(* Logix 5000 AddOnInstructionDefinition export Banner_IC70_Param_v4; software revision 33.03 *)

TYPE Banner_IC70_16P_Config_v4 :
STRUCT
   IO_Selection : INT;   // 0=NPN, 1=PNP
   Delay_Mode : INT;   // 0=Disabled,1=On Off Delay, 2=On OneShot, 3=Off OneShot, 4=On Pulse Stretcher, 5=Off Pulse Stretcher, 6=Totalizer, 7=Retriggerable On OneShot, 8=Retriggerable Off OneShot.
   Delay_Timer1 : DINT;
   Delay_Timer2 : DINT;
   Mirroring_Enable : SINT;   // 0=Disabled, 1=Enabled
   Mirroring_Channel : SINT;   // 0=C1, 1=C2, 2=C3, 3=C4, 4=C5, 5=C6, 6=C7, 7=C8, 8=C9, 9=C10, 10=C11, 11=C12, 12=C13, 13=C14, 14=C15, 15=C16
   Mirroring_Inversion : SINT;   // 0=Not Inverted, 1=Inverted
END_STRUCT
END_TYPE

TYPE Banner_IC70_16P_Direcrt_Param_v4 :
STRUCT
   Master_Cycle_Time : INT;
   Min_Cycle_Time : INT;
   M_Sequence_Capability : INT;
   IO_Link_Version_ID : INT;
   Process_Data_Input_Length : INT;
   Process_Data_Output_Length : INT;
   Combined_Vendor_ID : DINT;   // IO-Link Vendor ID
   Vendor_ID1 : INT;
   Vendor_ID2 : INT;
   Combined_Device_ID : DINT;   // IO-Link Device ID
   Device_ID1 : INT;
   Device_ID2 : INT;
   Device_ID3 : INT;
END_STRUCT
END_TYPE

TYPE Banner_IC70_16P_IO_Metrics_v4 :
STRUCT
   Count : DINT;
   Duration : DINT;
   Events_Per_Minute : DINT;
   Totalizer : DINT;
END_STRUCT
END_TYPE

TYPE Banner_IC70_16P_RD_v4 :   // UDT that stores the Write Data for a IC70-16P-K.
STRUCT
   Direct_Parameters : Banner_IC70_16P_Direcrt_Param_v4;
   Serial_Number : STRING;
   All_Time_Run_Time : DINT;   // Run Counter in 1/4 hr increments
   IO_Metrics : Banner_IC70_16P_IO_Metrics_v4[17];
END_STRUCT
END_TYPE

TYPE Banner_IC70_16P_SMR_Port_v4 :
STRUCT
   Reset : SINT;   // 0 = Normal setting, 1 = Reset metrics.
   Reset_Count : DINT;   // Value that Counter is set to when a Reset Metrics operation is activated.
END_STRUCT
END_TYPE

TYPE Banner_IC70_16P_v4 :   // All of the parameters for a IC70-16P.
STRUCT
   Initial_Global_Read : BOOL;   // Determines if all of the IO-Link data has been read into the PLC yet
   Command : INT;   // Value placed in here will activate a read or write to a specifc IO-Link Index
   Read : Banner_IC70_16P_RD_v4;   // Read Only Data
   Write : Banner_IC70_16P_WD_v4;   // Write Data
   Reset : BOOL;   // Resets AOI. This will force a complete parameter read of the sensor.
END_STRUCT
END_TYPE

TYPE Banner_IC70_16P_WD_v4 :   // UDT that stores the Write Data for a IC70-16P-K.
STRUCT
   System_Command : INT;   // See IODD file for list of commands that can be activated via the System Command interface
   Parameter_Access_Lock : SINT;   // Write access to all parameters is prohibited while value is 1. Only this parameter can be adjusted when value is 1.
   Data_Storage_Lock : SINT;   // Automatic data storage is disabled when this value is equal to 1. Read access is not affected.
   Local_Parameterization_Lock : SINT;   // Parameterization via local control elements on device is disabled.
   Local_User_Interface_Lock : SINT;   // Operation of local user interface is disabled.
   Resettable_Run_Time : DINT;   // Run Counter in 1/4 hr increments
   All_Time_Run_Time_Event_Time : DINT;   // Event Time in 1/4 hr increments
   Resettable_Run_Time_Event_Time : DINT;   // Event Time in 1/4 hour increments
   SMR : Banner_IC70_16P_SMR_Port_v4[17];   // Selectable Metric Reset.
   Channel_Config : Banner_IC70_16P_Config_v4[17];
END_STRUCT
END_TYPE

TYPE Banner_IOL_Port_v4 :   // UDT that has all of the data items necessary to communicate with a specific Port on a IO-Link Master
STRUCT
   Port_Controlled : INT;   // Each bit represents a port on an IO-Link Master. Set to 1 to tell AOI to control that port.
   Port_Activate : INT;   // Each bit represents a port on an IO-Link Master. When ON that port will process any commands in queue.
   Port_Read : INT;   // Each bit represents a port on an IO-Link Master. Used to determine when device AOI has requested a Read command.
   Port_Write : INT;   // Each bit represents a port on an IO-Link Master. Used to determine when device AOI has requested a Write command.
   Port_RW_Complete : INT;   // Each bit represents a port on an IO-Link Master. Tells device AOI that Read or Write request has been completed.
   Port_Device_Read : INT;
   Data_Transfer : SINT[190];   // Array to transfer data from IO-Master to device AOIs.
END_STRUCT
END_TYPE

ADD_ON_INSTRUCTION Banner_IC70_Param_v4   (* revision 4.4, vendor Banner Engineering *)
// AOI to read and write parameter data to an IC70-16P-K IO-Link Hub.
// Revision note:
// Added R130C.
VAR_IN_OUT
   Hub : Banner_IC70_16P_v4; {required}
   Port_Data : Banner_IOL_Port_v4; {required}
END_VAR
VAR_INPUT
   Port : INT; {required}
END_VAR
VAR
   Control : DINT; {access None}
   Global_Read_Command_Value : INT; {access None}
   Global_Write_Command_Value : INT; {access None}
   Command_Being_Processed : BOOL; {access None}
   Update_Archive : BOOL; {access None}
   Index_Write_Inprocess : INT; {access None}
   Index_Write_Control : INT; {access None}
   Temp_Excess_Gain : DINT; {access None}
   Inprocess_Index : DINT; {access None}
   Index2 : SINT; {access None}
   Index1 : SINT; {access None}
   Index4 : SINT; {access None}
   Index3 : SINT; {access None}
   Index6 : SINT; {access None}
   Index5 : SINT; {access None}
   Index7 : SINT; {access None}
END_VAR

ROUTINE Logic   (* ladder *)
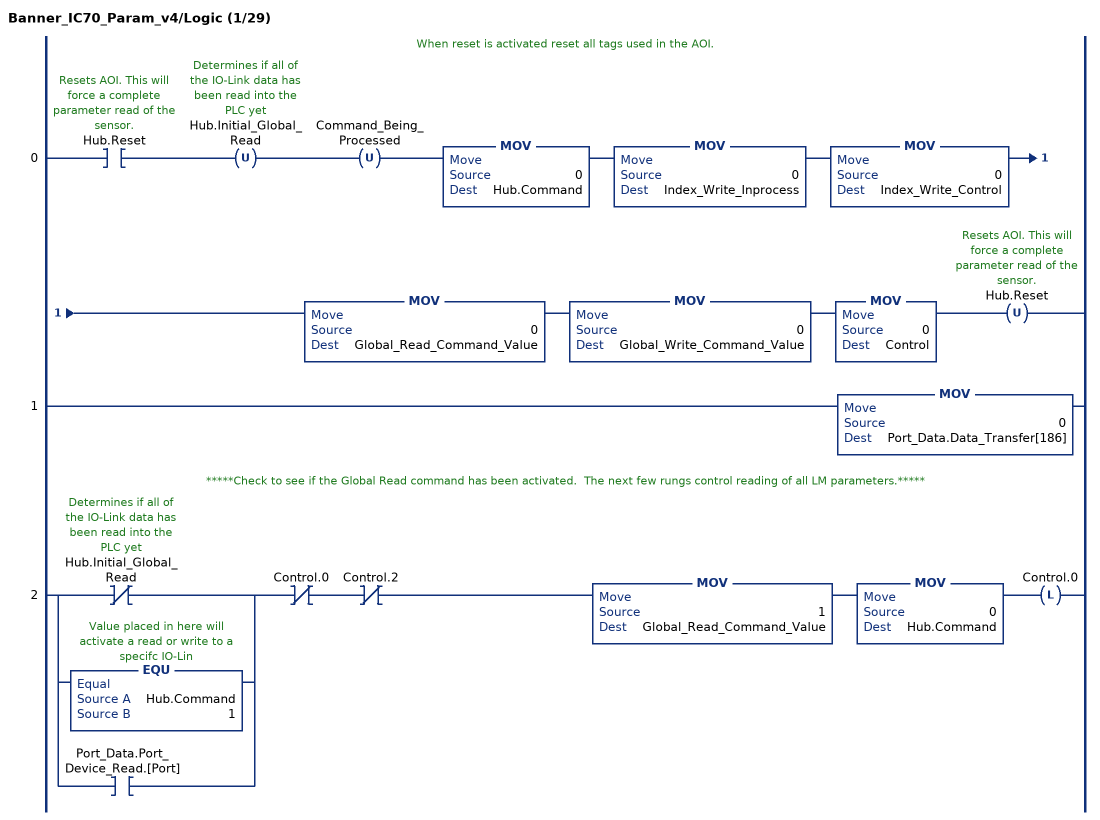
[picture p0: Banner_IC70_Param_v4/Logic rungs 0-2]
   // When reset is activated reset all tags used in the AOI.
   0: XIC(Hub.Reset)OTU(Hub.Initial_Global_Read)OTU(Command_Being_Processed)MOV(0,Hub.Command)MOV(0,Index_Write_Inprocess)MOV(0,Index_Write_Control)MOV(0,Global_Read_Command_Value)MOV(0,Global_Write_Command_Value)MOV(0,Control)OTU(Hub.Reset);
   1: MOV(0,Port_Data.Data_Transfer[186]);
   // *****Check to see if the Global Read command has been activated.  The next few rungs control reading of all LM parameters.*****
   2: [XIO(Hub.Initial_Global_Read) ,EQU(Hub.Command,1) ,XIC(Port_Data.Port_Device_Read.[Port]) ]XIO(Control.0)XIO(Control.2)MOV(1,Global_Read_Command_Value)MOV(0,Hub.Command)OTL(Control.0);
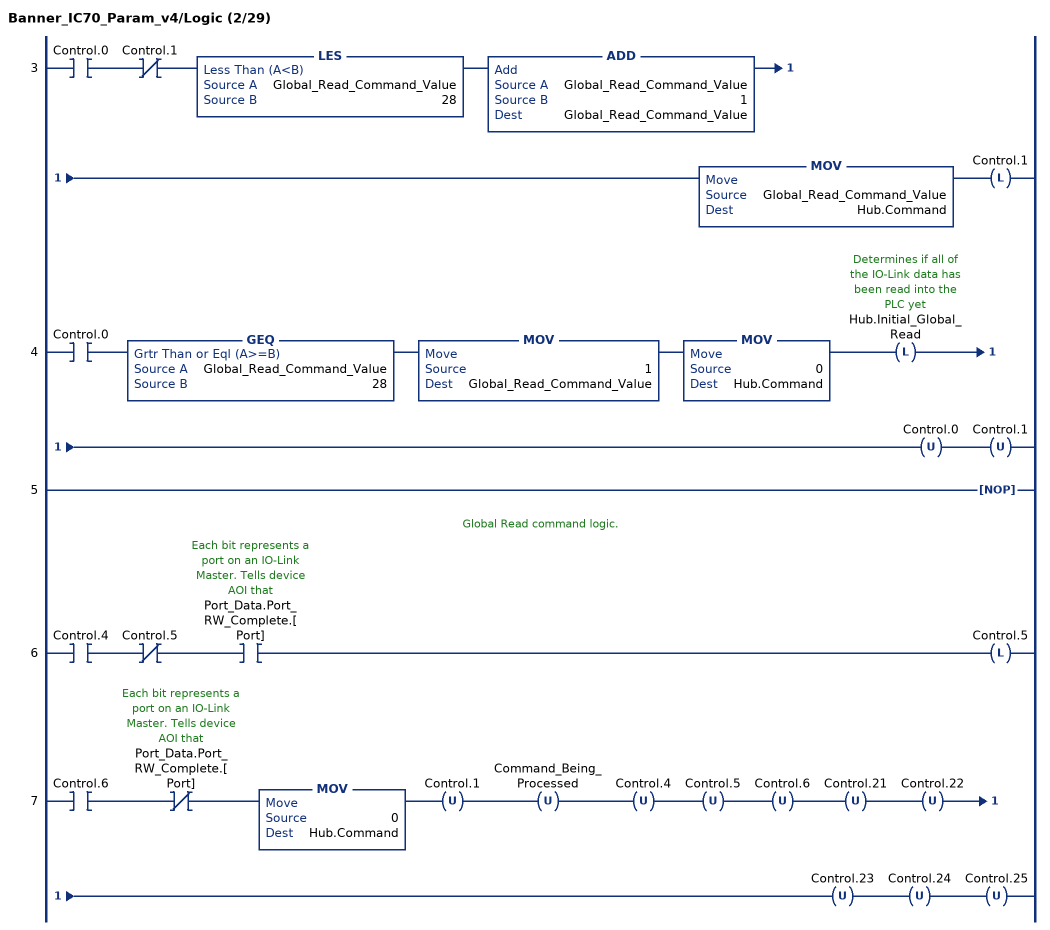
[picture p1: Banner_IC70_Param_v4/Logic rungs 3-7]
   3: XIC(Control.0)XIO(Control.1)LES(Global_Read_Command_Value,28)ADD(Global_Read_Command_Value,1,Global_Read_Command_Value)MOV(Global_Read_Command_Value,Hub.Command)OTL(Control.1);
   4: XIC(Control.0)GEQ(Global_Read_Command_Value,28)MOV(1,Global_Read_Command_Value)MOV(0,Hub.Command)OTL(Hub.Initial_Global_Read)OTU(Control.0)OTU(Control.1);
   5: NOP();
   // Global Read command logic.
   6: XIC(Control.4)XIO(Control.5)XIC(Port_Data.Port_RW_Complete.[Port])OTL(Control.5);
   7: XIC(Control.6)XIO(Port_Data.Port_RW_Complete.[Port])MOV(0,Hub.Command)OTU(Control.1)OTU(Command_Being_Processed)OTU(Control.4)OTU(Control.5)OTU(Control.6)OTU(Control.21)OTU(Control.22)OTU(Control.23)OTU(Control.24)OTU(Control.25);
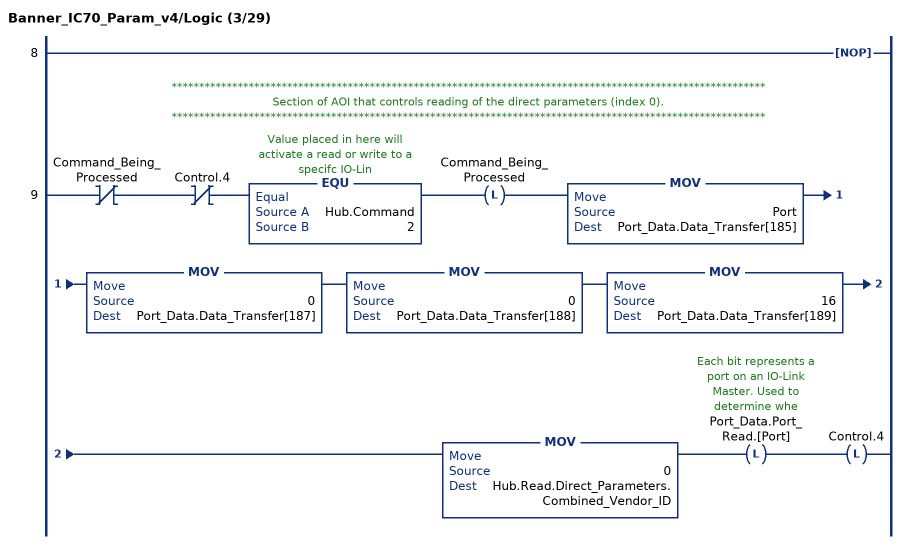
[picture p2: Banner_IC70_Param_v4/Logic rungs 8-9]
   8: NOP();
   // ************************************************************************************************************
   // Section of AOI that controls reading of the direct parameters (index 0).
   // ************************************************************************************************************
   9: XIO(Command_Being_Processed)XIO(Control.4)EQU(Hub.Command,2)OTL(Command_Being_Processed)MOV(Port,Port_Data.Data_Transfer[185])MOV(0,Port_Data.Data_Transfer[187])MOV(0,Port_Data.Data_Transfer[188])MOV(16,Port_Data.Data_Transfer[189])MOV(0,Hub.Read.Direct_Parameters.Combined_Vendor_ID)OTL(Port_Data.Port_Read.[Port])OTL(Control.4);
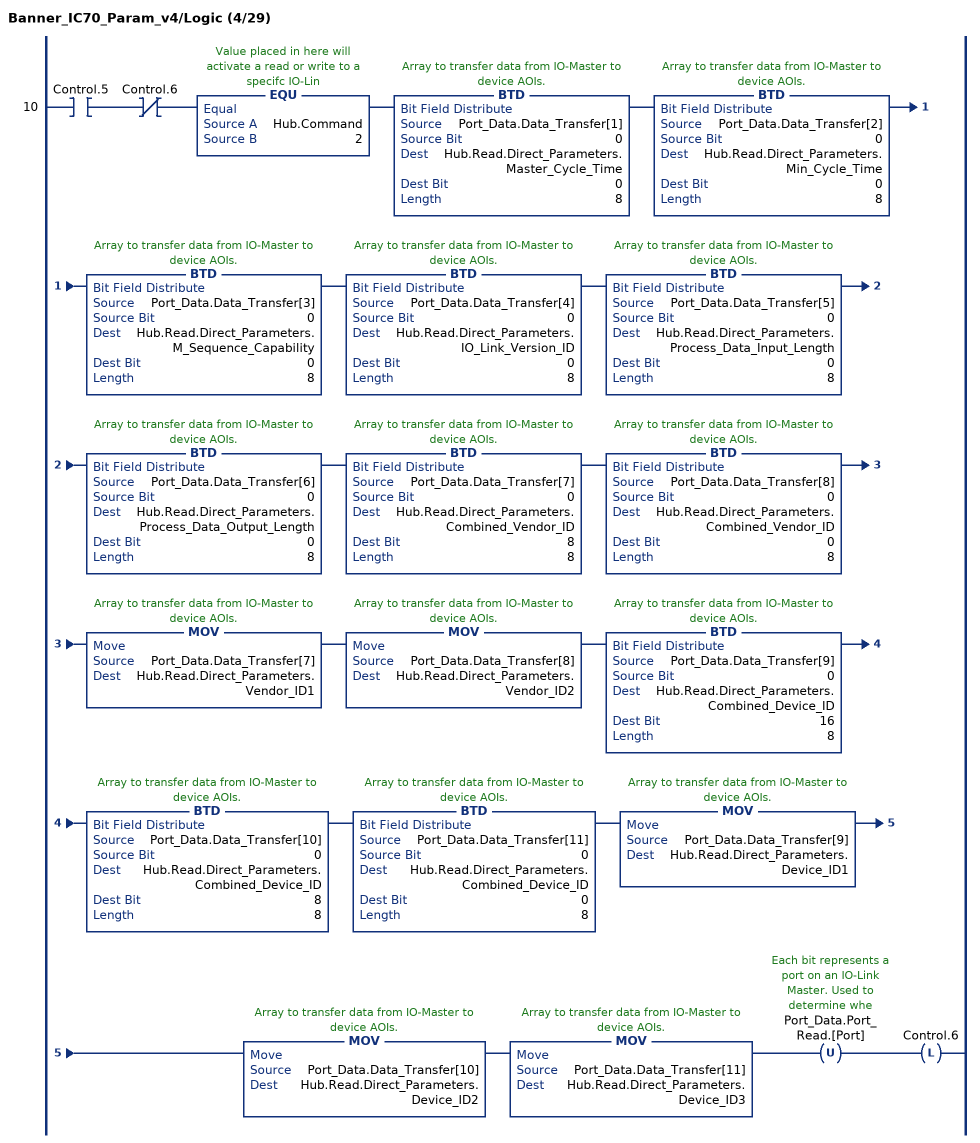
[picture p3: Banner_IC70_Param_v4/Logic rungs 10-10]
   10: XIC(Control.5)XIO(Control.6)EQU(Hub.Command,2)BTD(Port_Data.Data_Transfer[1],0,Hub.Read.Direct_Parameters.Master_Cycle_Time,0,8)BTD(Port_Data.Data_Transfer[2],0,Hub.Read.Direct_Parameters.Min_Cycle_Time,0,8)BTD(Port_Data.Data_Transfer[3],0,Hub.Read.Direct_Parameters.M_Sequence_Capability,0,8)BTD(Port_Data.Data_Transfer[4],0,Hub.Read.Direct_Parameters.IO_Link_Version_ID,0,8)BTD(Port_Data.Data_Transfer[5],0,Hub.Read.Direct_Parameters.Process_Data_Input_Length,0,8)BTD(Port_Data.Data_Transfer[6],0,Hub.Read.Direct_Parameters.Process_Data_Output_Length,0,8)BTD(Port_Data.Data_Transfer[7],0,Hub.Read.Direct_Parameters.Combined_Vendor_ID,8,8)BTD(Port_Data.Data_Transfer[8],0,Hub.Read.Direct_Parameters.Combined_Vendor_ID,0,8)MOV(Port_Data.Data_Transfer[7],Hub.Read.Direct_Parameters.Vendor_ID1)MOV(Port_Data.Data_Transfer[8],Hub.Read.Direct_Parameters.Vendor_ID2)BTD(Port_Data.Data_Transfer[9],0,Hub.Read.Direct_Parameters.Combined_Device_ID,16,8)BTD(Port_Data.Data_Transfer[10],0,Hub.Read.Direct_Parameters.Combined_Device_ID,8,8)BTD(Port_Data.Data_Transfer[11],0,Hub.Read.Direct_Parameters.Combined_Device_ID,0,8)MOV(Port_Data.Data_Transfer[9],Hub.Read.Direct_Parameters.Device_ID1)MOV(Port_Data.Data_Transfer[10],Hub.Read.Direct_Parameters.Device_ID2)MOV(Port_Data.Data_Transfer[11],Hub.Read.Direct_Parameters.Device_ID3)OTU(Port_Data.Port_Read.[Port])OTL(Control.6);
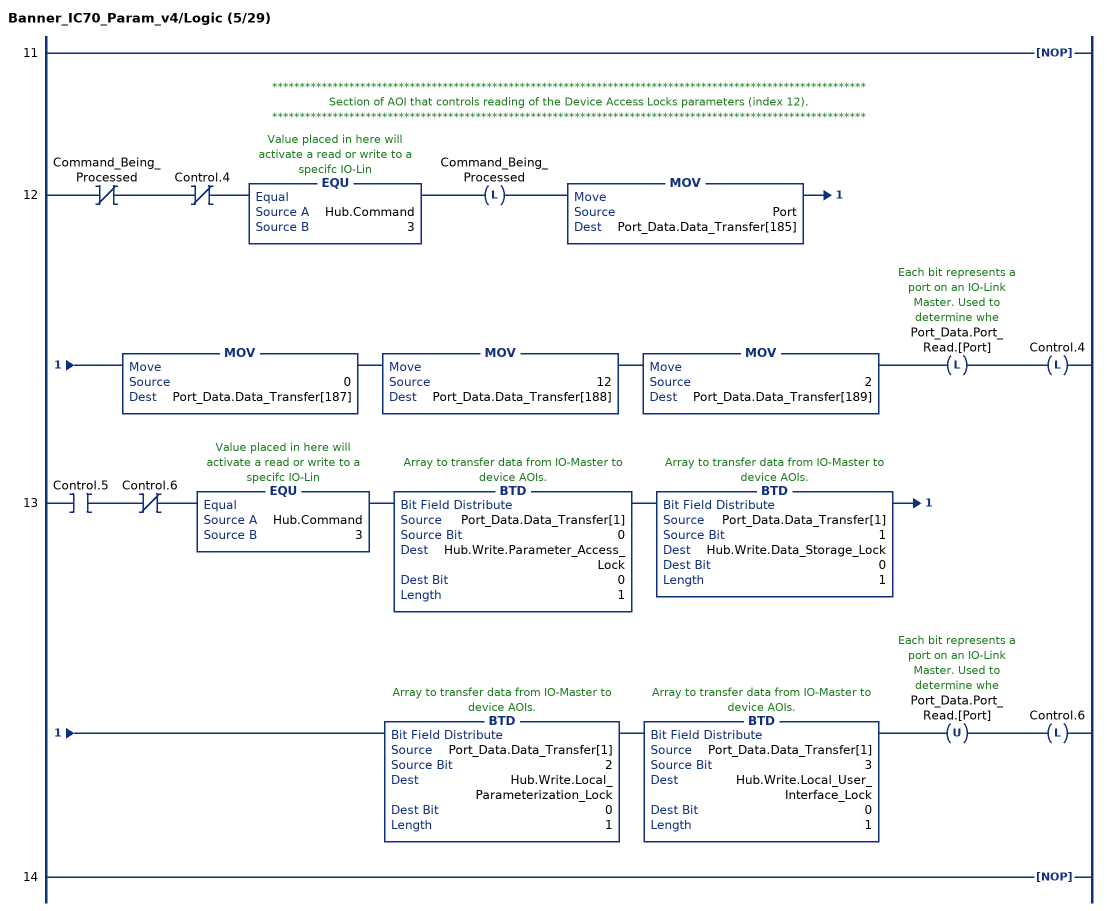
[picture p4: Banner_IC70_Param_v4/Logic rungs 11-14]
   11: NOP();
   // ************************************************************************************************************
   // Section of AOI that controls reading of the Device Access Locks parameters (index 12).
   // ************************************************************************************************************
   12: XIO(Command_Being_Processed)XIO(Control.4)EQU(Hub.Command,3)OTL(Command_Being_Processed)MOV(Port,Port_Data.Data_Transfer[185])MOV(0,Port_Data.Data_Transfer[187])MOV(12,Port_Data.Data_Transfer[188])MOV(2,Port_Data.Data_Transfer[189])OTL(Port_Data.Port_Read.[Port])OTL(Control.4);
   13: XIC(Control.5)XIO(Control.6)EQU(Hub.Command,3)BTD(Port_Data.Data_Transfer[1],0,Hub.Write.Parameter_Access_Lock,0,1)BTD(Port_Data.Data_Transfer[1],1,Hub.Write.Data_Storage_Lock,0,1)BTD(Port_Data.Data_Transfer[1],2,Hub.Write.Local_Parameterization_Lock,0,1)BTD(Port_Data.Data_Transfer[1],3,Hub.Write.Local_User_Interface_Lock,0,1)OTU(Port_Data.Port_Read.[Port])OTL(Control.6);
   14: NOP();
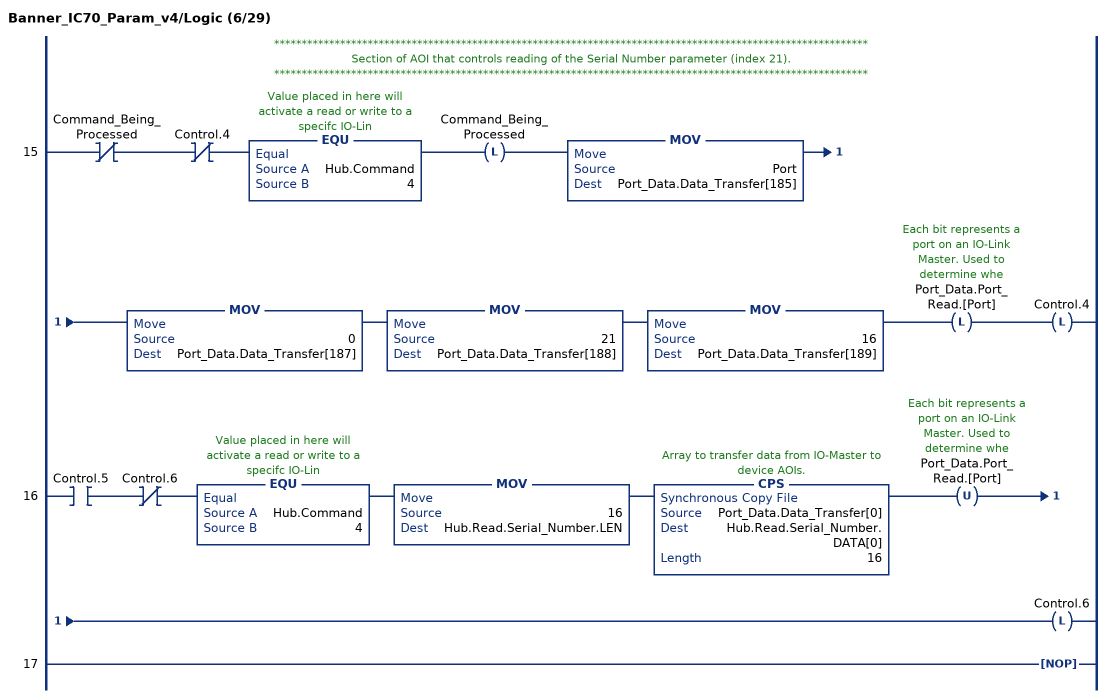
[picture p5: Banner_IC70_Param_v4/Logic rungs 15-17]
   // ************************************************************************************************************
   // Section of AOI that controls reading of the Serial Number parameter (index 21).
   // ************************************************************************************************************
   15: XIO(Command_Being_Processed)XIO(Control.4)EQU(Hub.Command,4)OTL(Command_Being_Processed)MOV(Port,Port_Data.Data_Transfer[185])MOV(0,Port_Data.Data_Transfer[187])MOV(21,Port_Data.Data_Transfer[188])MOV(16,Port_Data.Data_Transfer[189])OTL(Port_Data.Port_Read.[Port])OTL(Control.4);
   16: XIC(Control.5)XIO(Control.6)EQU(Hub.Command,4)MOV(16,Hub.Read.Serial_Number.LEN)CPS(Port_Data.Data_Transfer[0],Hub.Read.Serial_Number.DATA[0],16)OTU(Port_Data.Port_Read.[Port])OTL(Control.6);
   17: NOP();
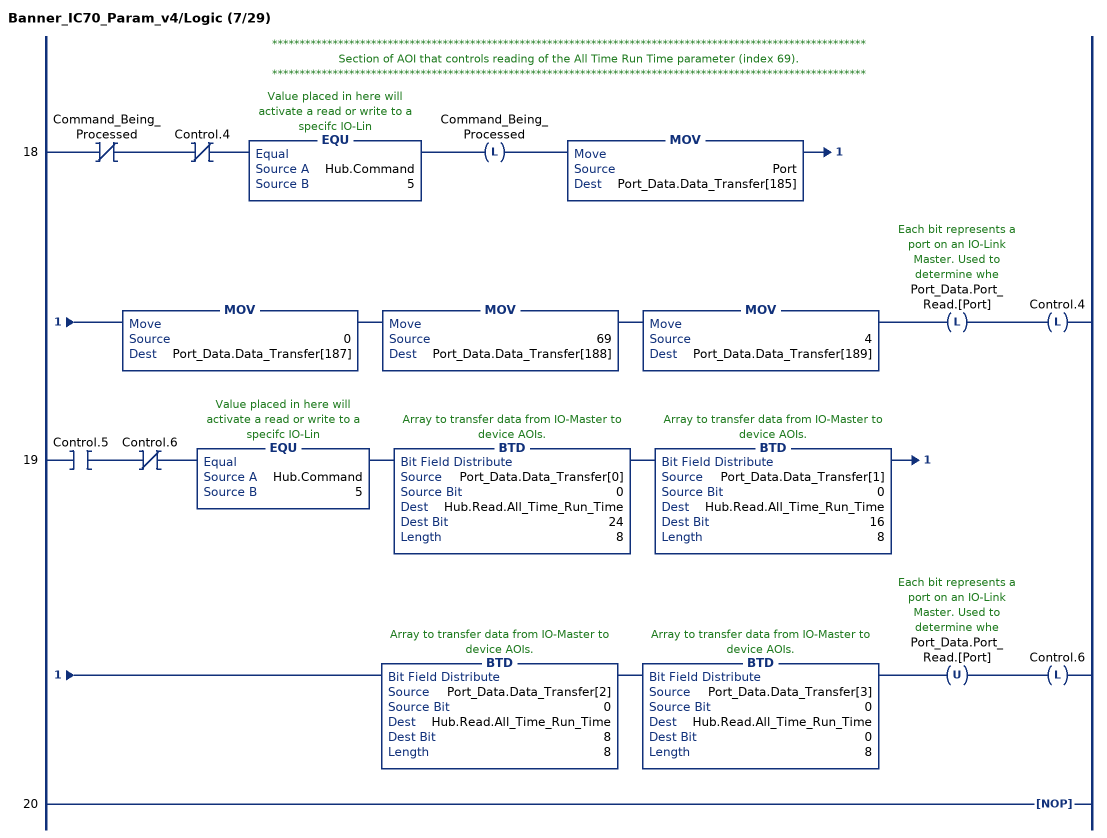
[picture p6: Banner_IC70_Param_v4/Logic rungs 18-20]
   // ************************************************************************************************************
   // Section of AOI that controls reading of the All Time Run Time parameter (index 69).
   // ************************************************************************************************************
   18: XIO(Command_Being_Processed)XIO(Control.4)EQU(Hub.Command,5)OTL(Command_Being_Processed)MOV(Port,Port_Data.Data_Transfer[185])MOV(0,Port_Data.Data_Transfer[187])MOV(69,Port_Data.Data_Transfer[188])MOV(4,Port_Data.Data_Transfer[189])OTL(Port_Data.Port_Read.[Port])OTL(Control.4);
   19: XIC(Control.5)XIO(Control.6)EQU(Hub.Command,5)BTD(Port_Data.Data_Transfer[0],0,Hub.Read.All_Time_Run_Time,24,8)BTD(Port_Data.Data_Transfer[1],0,Hub.Read.All_Time_Run_Time,16,8)BTD(Port_Data.Data_Transfer[2],0,Hub.Read.All_Time_Run_Time,8,8)BTD(Port_Data.Data_Transfer[3],0,Hub.Read.All_Time_Run_Time,0,8)OTU(Port_Data.Port_Read.[Port])OTL(Control.6);
   20: NOP();
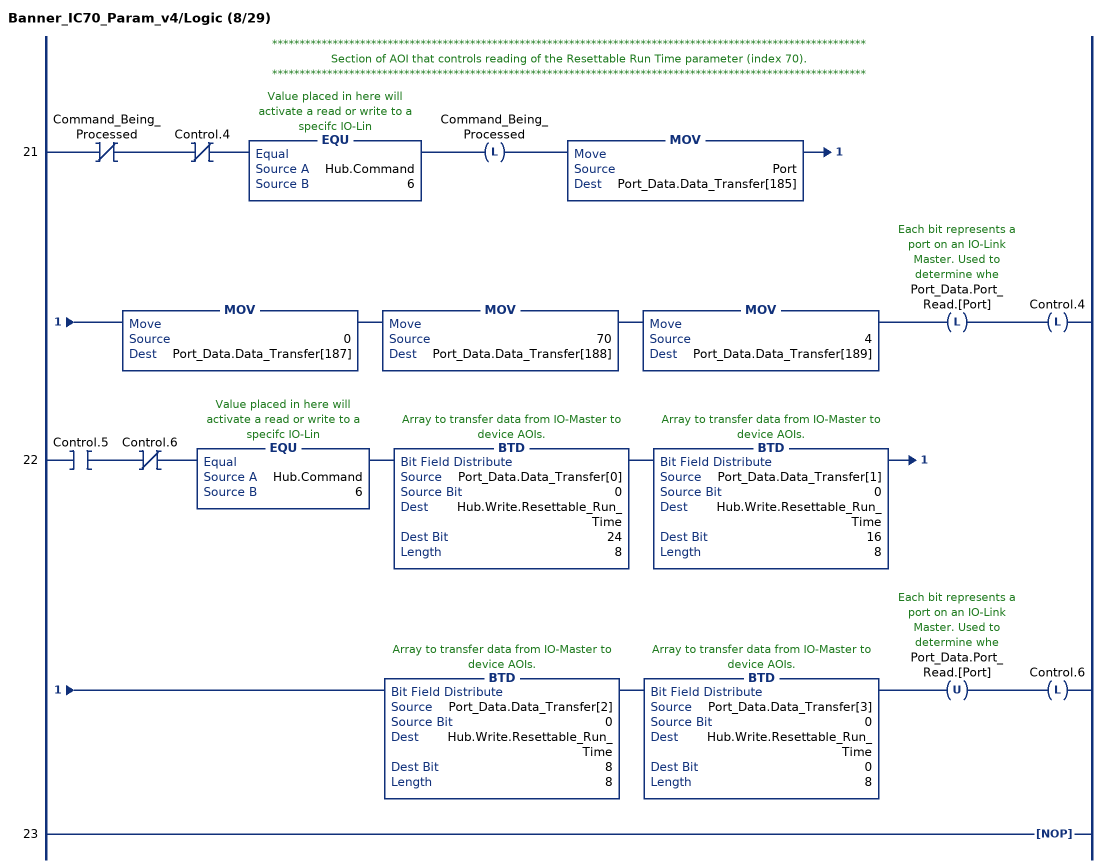
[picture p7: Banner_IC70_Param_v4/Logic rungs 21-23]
   // ************************************************************************************************************
   // Section of AOI that controls reading of the Resettable Run Time parameter (index 70).
   // ************************************************************************************************************
   21: XIO(Command_Being_Processed)XIO(Control.4)EQU(Hub.Command,6)OTL(Command_Being_Processed)MOV(Port,Port_Data.Data_Transfer[185])MOV(0,Port_Data.Data_Transfer[187])MOV(70,Port_Data.Data_Transfer[188])MOV(4,Port_Data.Data_Transfer[189])OTL(Port_Data.Port_Read.[Port])OTL(Control.4);
   22: XIC(Control.5)XIO(Control.6)EQU(Hub.Command,6)BTD(Port_Data.Data_Transfer[0],0,Hub.Write.Resettable_Run_Time,24,8)BTD(Port_Data.Data_Transfer[1],0,Hub.Write.Resettable_Run_Time,16,8)BTD(Port_Data.Data_Transfer[2],0,Hub.Write.Resettable_Run_Time,8,8)BTD(Port_Data.Data_Transfer[3],0,Hub.Write.Resettable_Run_Time,0,8)OTU(Port_Data.Port_Read.[Port])OTL(Control.6);
   23: NOP();
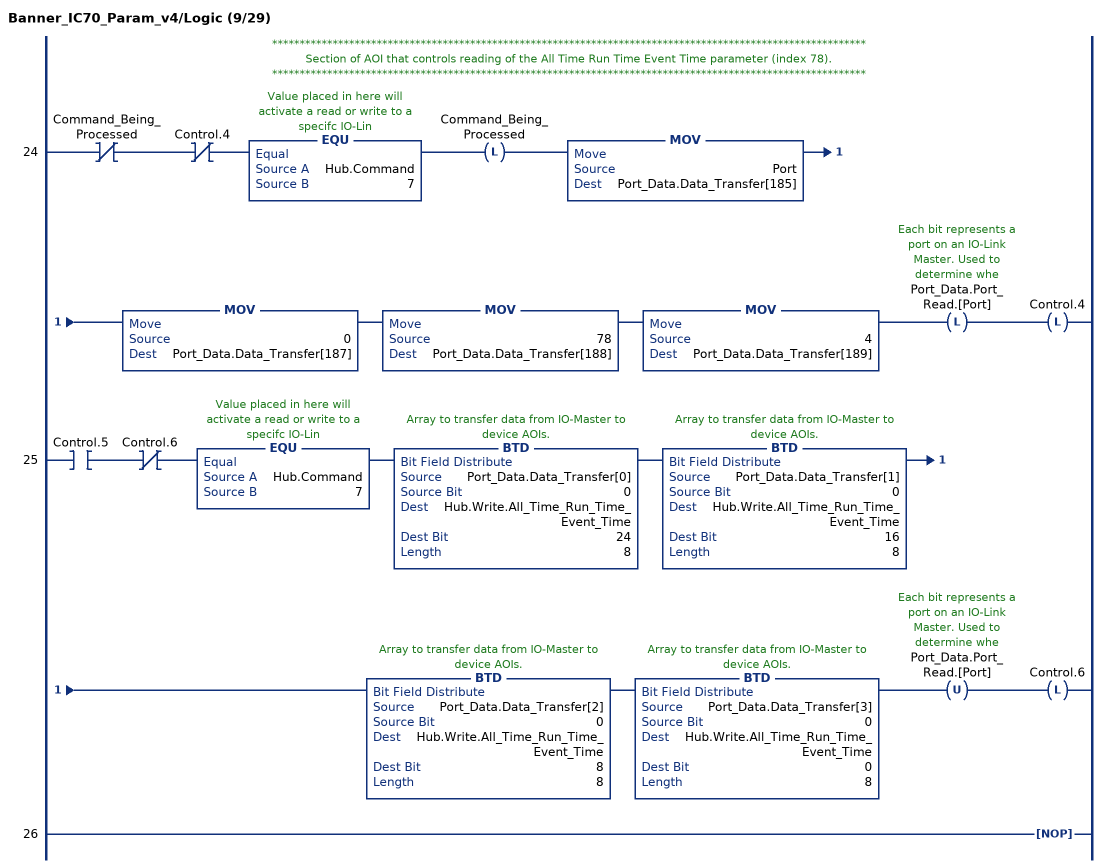
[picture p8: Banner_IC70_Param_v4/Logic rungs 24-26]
   // ************************************************************************************************************
   // Section of AOI that controls reading of the All Time Run Time Event Time parameter (index 78).
   // ************************************************************************************************************
   24: XIO(Command_Being_Processed)XIO(Control.4)EQU(Hub.Command,7)OTL(Command_Being_Processed)MOV(Port,Port_Data.Data_Transfer[185])MOV(0,Port_Data.Data_Transfer[187])MOV(78,Port_Data.Data_Transfer[188])MOV(4,Port_Data.Data_Transfer[189])OTL(Port_Data.Port_Read.[Port])OTL(Control.4);
   25: XIC(Control.5)XIO(Control.6)EQU(Hub.Command,7)BTD(Port_Data.Data_Transfer[0],0,Hub.Write.All_Time_Run_Time_Event_Time,24,8)BTD(Port_Data.Data_Transfer[1],0,Hub.Write.All_Time_Run_Time_Event_Time,16,8)BTD(Port_Data.Data_Transfer[2],0,Hub.Write.All_Time_Run_Time_Event_Time,8,8)BTD(Port_Data.Data_Transfer[3],0,Hub.Write.All_Time_Run_Time_Event_Time,0,8)OTU(Port_Data.Port_Read.[Port])OTL(Control.6);
   26: NOP();
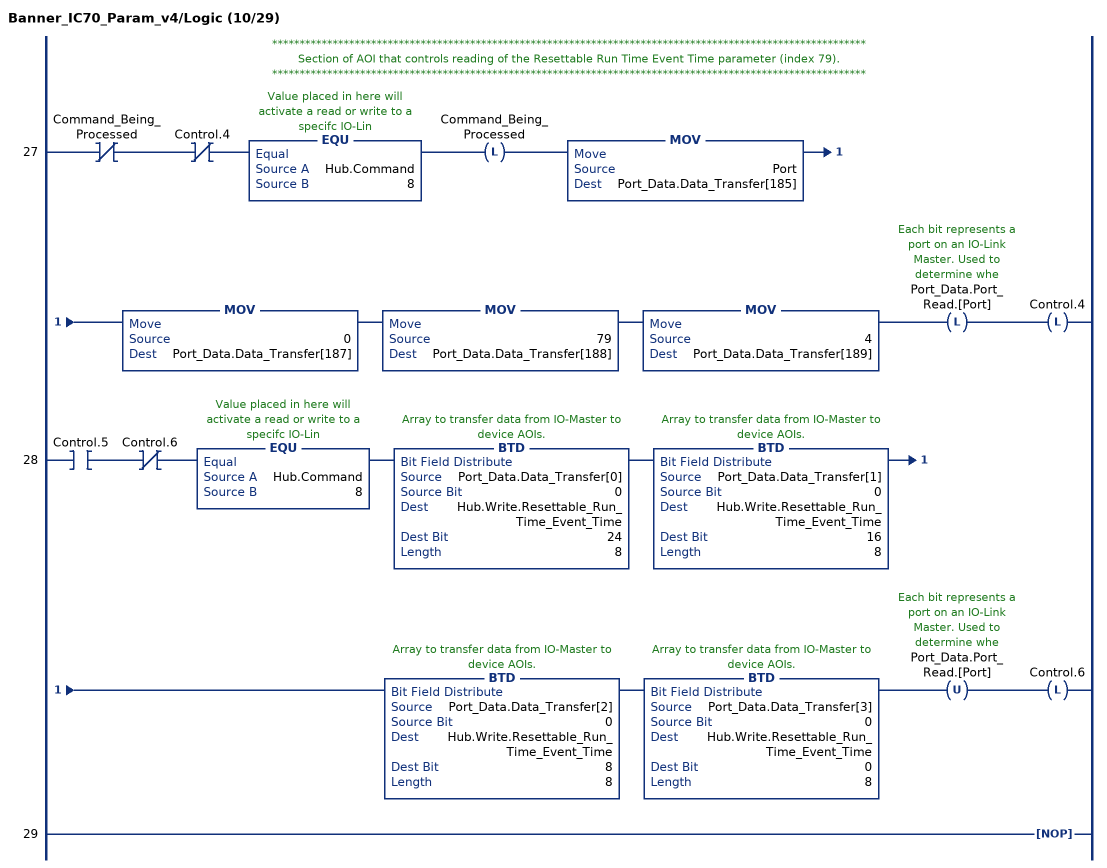
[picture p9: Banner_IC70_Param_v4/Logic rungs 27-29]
   // ************************************************************************************************************
   // Section of AOI that controls reading of the Resettable Run Time Event Time parameter (index 79).
   // ************************************************************************************************************
   27: XIO(Command_Being_Processed)XIO(Control.4)EQU(Hub.Command,8)OTL(Command_Being_Processed)MOV(Port,Port_Data.Data_Transfer[185])MOV(0,Port_Data.Data_Transfer[187])MOV(79,Port_Data.Data_Transfer[188])MOV(4,Port_Data.Data_Transfer[189])OTL(Port_Data.Port_Read.[Port])OTL(Control.4);
   28: XIC(Control.5)XIO(Control.6)EQU(Hub.Command,8)BTD(Port_Data.Data_Transfer[0],0,Hub.Write.Resettable_Run_Time_Event_Time,24,8)BTD(Port_Data.Data_Transfer[1],0,Hub.Write.Resettable_Run_Time_Event_Time,16,8)BTD(Port_Data.Data_Transfer[2],0,Hub.Write.Resettable_Run_Time_Event_Time,8,8)BTD(Port_Data.Data_Transfer[3],0,Hub.Write.Resettable_Run_Time_Event_Time,0,8)OTU(Port_Data.Port_Read.[Port])OTL(Control.6);
   29: NOP();
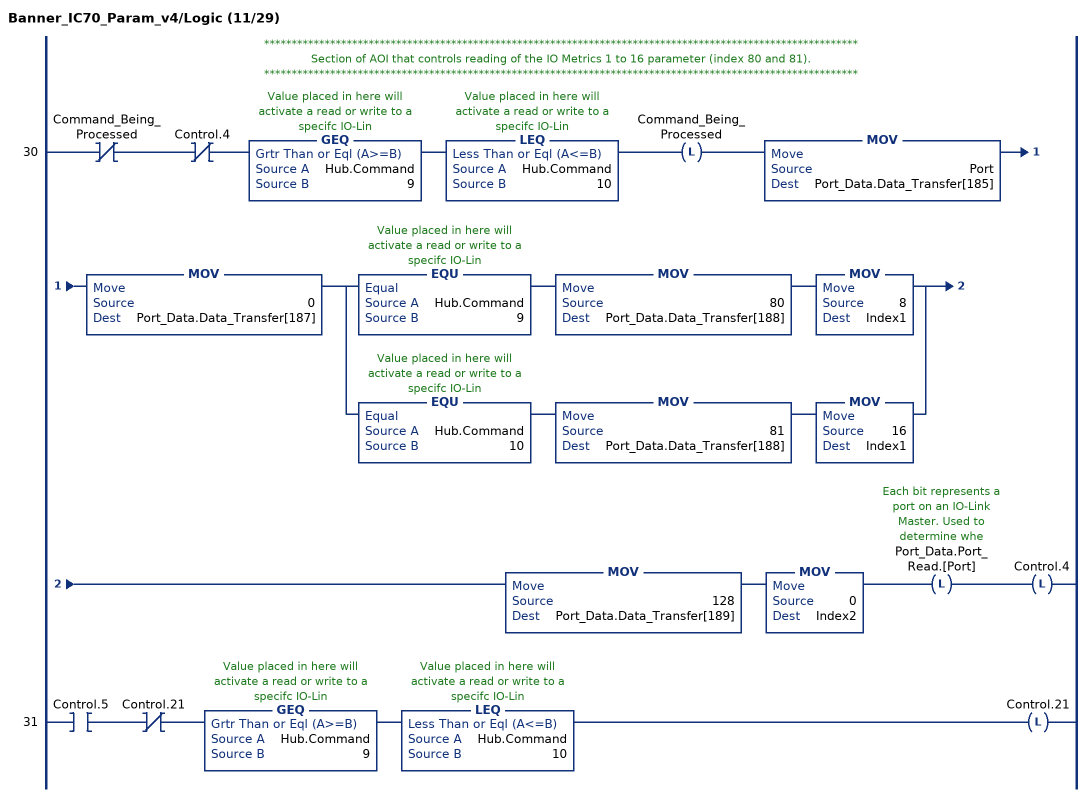
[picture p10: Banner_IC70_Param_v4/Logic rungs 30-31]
   // ************************************************************************************************************
   // Section of AOI that controls reading of the IO Metrics 1 to 16 parameter (index 80 and 81).
   // ************************************************************************************************************
   30: XIO(Command_Being_Processed)XIO(Control.4)GEQ(Hub.Command,9)LEQ(Hub.Command,10)OTL(Command_Being_Processed)MOV(Port,Port_Data.Data_Transfer[185])MOV(0,Port_Data.Data_Transfer[187])[EQU(Hub.Command,9) MOV(80,Port_Data.Data_Transfer[188]) MOV(8,Index1) ,EQU(Hub.Command,10) MOV(81,Port_Data.Data_Transfer[188]) MOV(16,Index1) ]MOV(128,Port_Data.Data_Transfer[189])MOV(0,Index2)OTL(Port_Data.Port_Read.[Port])OTL(Control.4);
   31: XIC(Control.5)XIO(Control.21)GEQ(Hub.Command,9)LEQ(Hub.Command,10)OTL(Control.21);
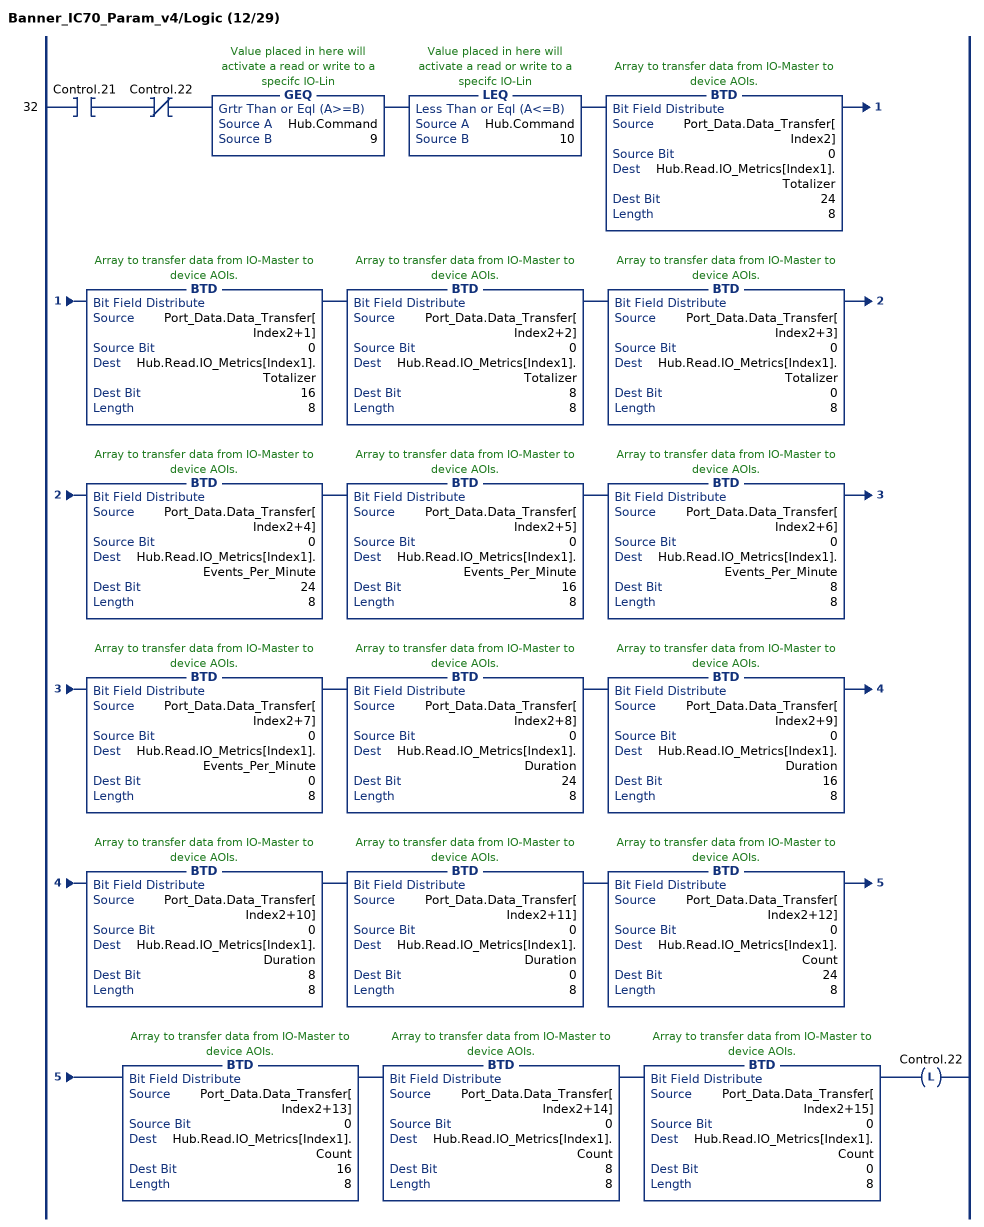
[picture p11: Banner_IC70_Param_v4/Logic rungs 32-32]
   32: XIC(Control.21)XIO(Control.22)GEQ(Hub.Command,9)LEQ(Hub.Command,10)BTD(Port_Data.Data_Transfer[Index2],0,Hub.Read.IO_Metrics[Index1].Totalizer,24,8)BTD(Port_Data.Data_Transfer[Index2+1],0,Hub.Read.IO_Metrics[Index1].Totalizer,16,8)BTD(Port_Data.Data_Transfer[Index2+2],0,Hub.Read.IO_Metrics[Index1].Totalizer,8,8)BTD(Port_Data.Data_Transfer[Index2+3],0,Hub.Read.IO_Metrics[Index1].Totalizer,0,8)BTD(Port_Data.Data_Transfer[Index2+4],0,Hub.Read.IO_Metrics[Index1].Events_Per_Minute,24,8)BTD(Port_Data.Data_Transfer[Index2+5],0,Hub.Read.IO_Metrics[Index1].Events_Per_Minute,16,8)BTD(Port_Data.Data_Transfer[Index2+6],0,Hub.Read.IO_Metrics[Index1].Events_Per_Minute,8,8)BTD(Port_Data.Data_Transfer[Index2+7],0,Hub.Read.IO_Metrics[Index1].Events_Per_Minute,0,8)BTD(Port_Data.Data_Transfer[Index2+8],0,Hub.Read.IO_Metrics[Index1].Duration,24,8)BTD(Port_Data.Data_Transfer[Index2+9],0,Hub.Read.IO_Metrics[Index1].Duration,16,8)BTD(Port_Data.Data_Transfer[Index2+10],0,Hub.Read.IO_Metrics[Index1].Duration,8,8)BTD(Port_Data.Data_Transfer[Index2+11],0,Hub.Read.IO_Metrics[Index1].Duration,0,8)BTD(Port_Data.Data_Transfer[Index2+12],0,Hub.Read.IO_Metrics[Index1].Count,24,8)BTD(Port_Data.Data_Transfer[Index2+13],0,Hub.Read.IO_Metrics[Index1].Count,16,8)BTD(Port_Data.Data_Transfer[Index2+14],0,Hub.Read.IO_Metrics[Index1].Count,8,8)BTD(Port_Data.Data_Transfer[Index2+15],0,Hub.Read.IO_Metrics[Index1].Count,0,8)OTL(Control.22);
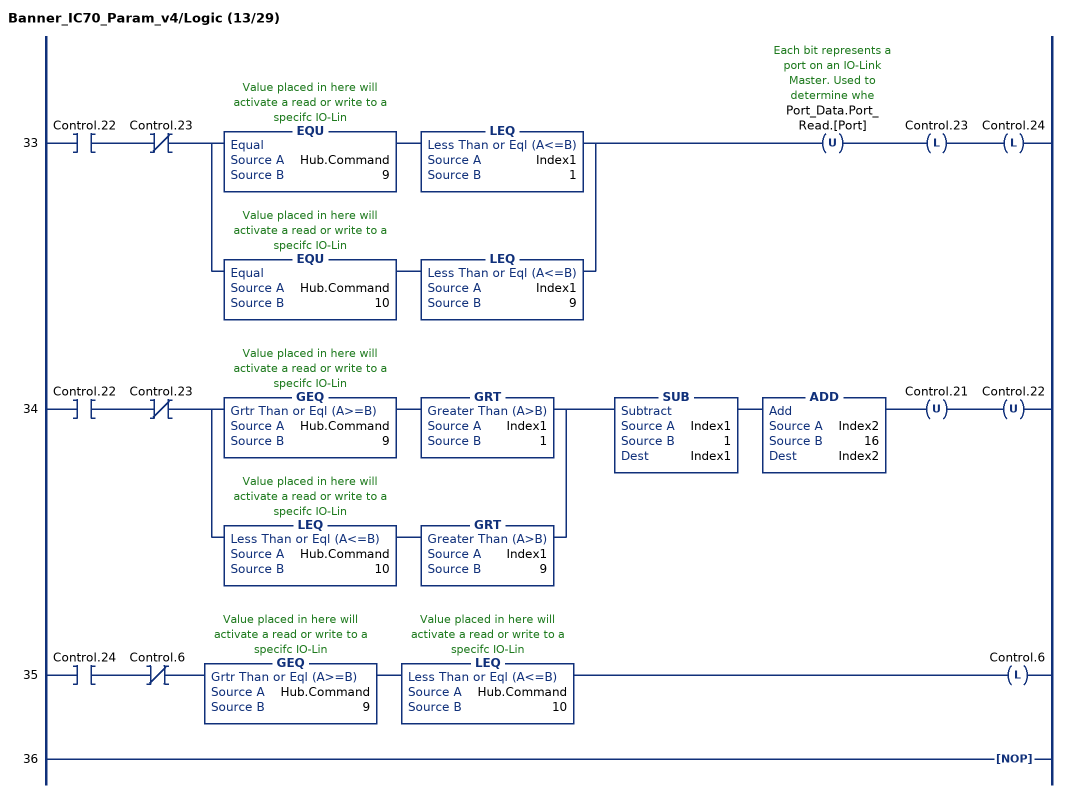
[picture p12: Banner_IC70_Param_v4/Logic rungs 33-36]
   33: XIC(Control.22)XIO(Control.23)[EQU(Hub.Command,9) LEQ(Index1,1) ,EQU(Hub.Command,10) LEQ(Index1,9) ]OTU(Port_Data.Port_Read.[Port])OTL(Control.23)OTL(Control.24);
   34: XIC(Control.22)XIO(Control.23)[GEQ(Hub.Command,9) GRT(Index1,1) ,LEQ(Hub.Command,10) GRT(Index1,9) ]SUB(Index1,1,Index1)ADD(Index2,16,Index2)OTU(Control.21)OTU(Control.22);
   35: XIC(Control.24)XIO(Control.6)GEQ(Hub.Command,9)LEQ(Hub.Command,10)OTL(Control.6);
   36: NOP();
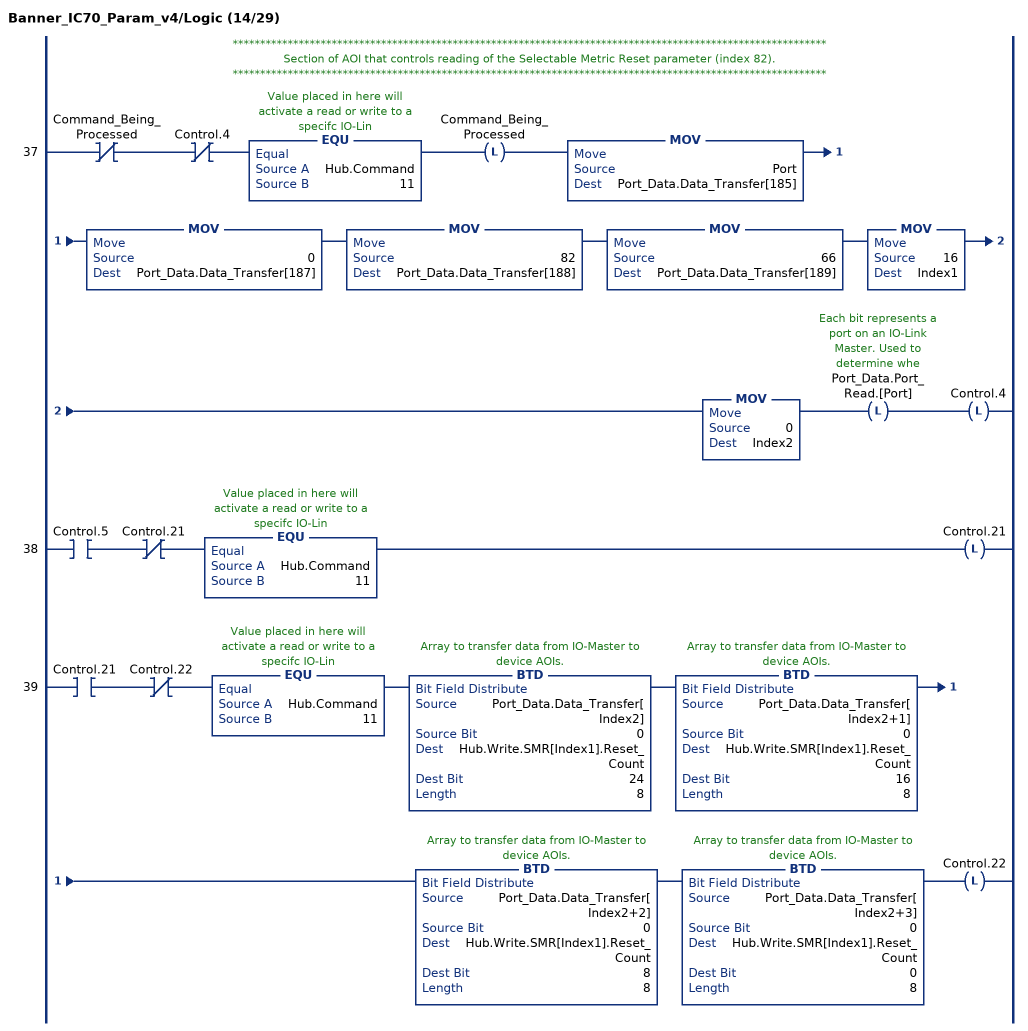
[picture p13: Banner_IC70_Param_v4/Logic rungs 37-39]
   // ************************************************************************************************************
   // Section of AOI that controls reading of the Selectable Metric Reset parameter (index 82).
   // ************************************************************************************************************
   37: XIO(Command_Being_Processed)XIO(Control.4)EQU(Hub.Command,11)OTL(Command_Being_Processed)MOV(Port,Port_Data.Data_Transfer[185])MOV(0,Port_Data.Data_Transfer[187])MOV(82,Port_Data.Data_Transfer[188])MOV(66,Port_Data.Data_Transfer[189])MOV(16,Index1)MOV(0,Index2)OTL(Port_Data.Port_Read.[Port])OTL(Control.4);
   38: XIC(Control.5)XIO(Control.21)EQU(Hub.Command,11)OTL(Control.21);
   39: XIC(Control.21)XIO(Control.22)EQU(Hub.Command,11)BTD(Port_Data.Data_Transfer[Index2],0,Hub.Write.SMR[Index1].Reset_Count,24,8)BTD(Port_Data.Data_Transfer[Index2+1],0,Hub.Write.SMR[Index1].Reset_Count,16,8)BTD(Port_Data.Data_Transfer[Index2+2],0,Hub.Write.SMR[Index1].Reset_Count,8,8)BTD(Port_Data.Data_Transfer[Index2+3],0,Hub.Write.SMR[Index1].Reset_Count,0,8)OTL(Control.22);
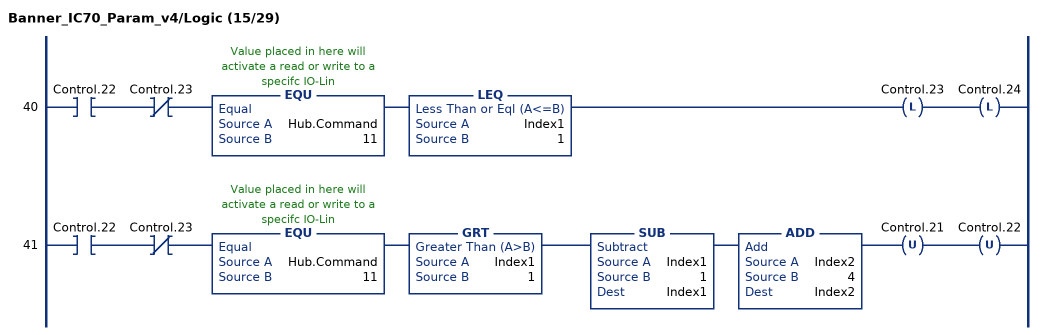
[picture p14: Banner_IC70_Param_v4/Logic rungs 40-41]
   40: XIC(Control.22)XIO(Control.23)EQU(Hub.Command,11)LEQ(Index1,1)OTL(Control.23)OTL(Control.24);
   41: XIC(Control.22)XIO(Control.23)EQU(Hub.Command,11)GRT(Index1,1)SUB(Index1,1,Index1)ADD(Index2,4,Index2)OTU(Control.21)OTU(Control.22);
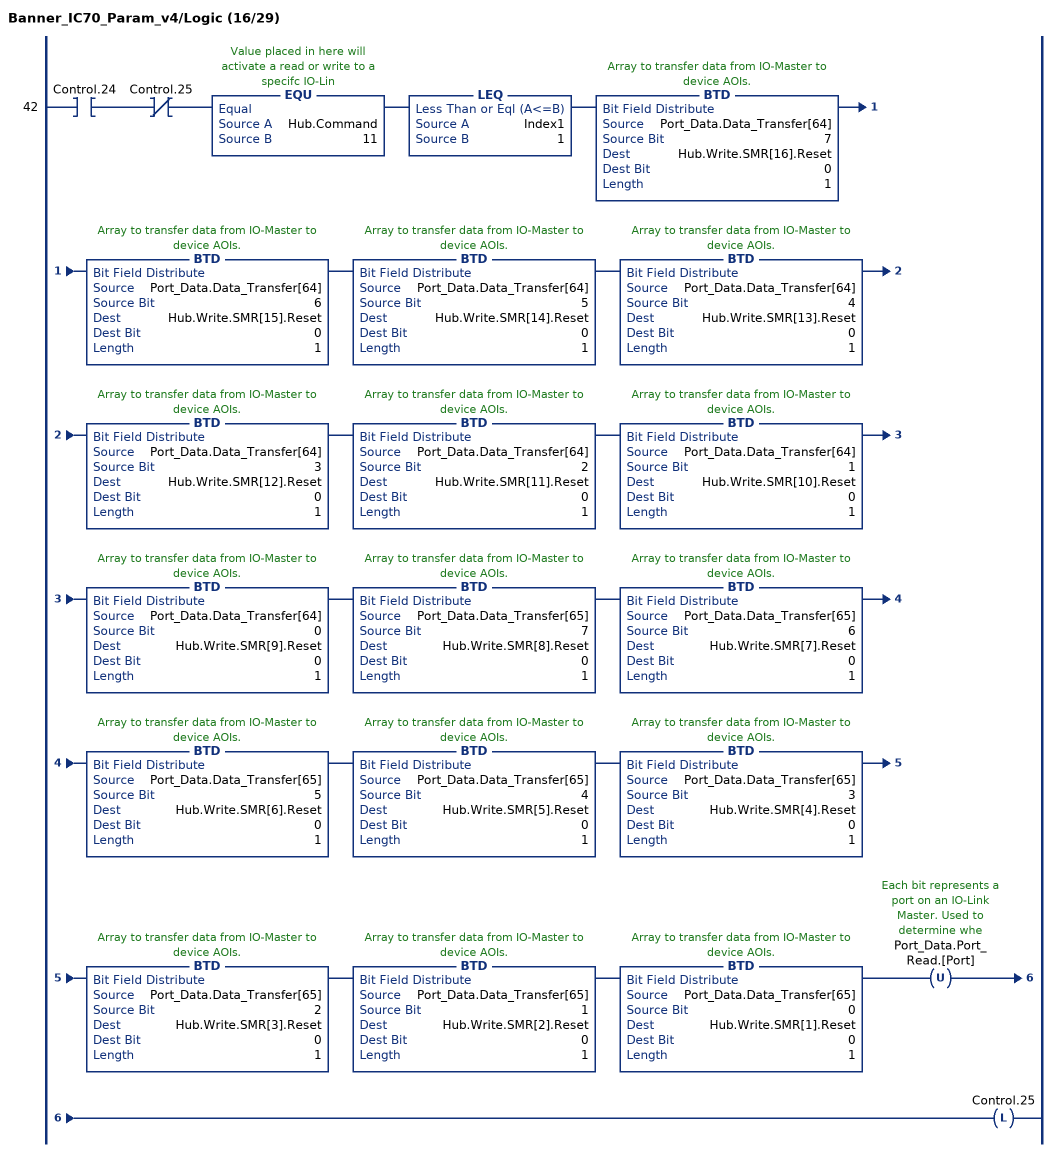
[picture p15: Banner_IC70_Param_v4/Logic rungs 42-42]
   42: XIC(Control.24)XIO(Control.25)EQU(Hub.Command,11)LEQ(Index1,1)BTD(Port_Data.Data_Transfer[64],7,Hub.Write.SMR[16].Reset,0,1)BTD(Port_Data.Data_Transfer[64],6,Hub.Write.SMR[15].Reset,0,1)BTD(Port_Data.Data_Transfer[64],5,Hub.Write.SMR[14].Reset,0,1)BTD(Port_Data.Data_Transfer[64],4,Hub.Write.SMR[13].Reset,0,1)BTD(Port_Data.Data_Transfer[64],3,Hub.Write.SMR[12].Reset,0,1)BTD(Port_Data.Data_Transfer[64],2,Hub.Write.SMR[11].Reset,0,1)BTD(Port_Data.Data_Transfer[64],1,Hub.Write.SMR[10].Reset,0,1)BTD(Port_Data.Data_Transfer[64],0,Hub.Write.SMR[9].Reset,0,1)BTD(Port_Data.Data_Transfer[65],7,Hub.Write.SMR[8].Reset,0,1)BTD(Port_Data.Data_Transfer[65],6,Hub.Write.SMR[7].Reset,0,1)BTD(Port_Data.Data_Transfer[65],5,Hub.Write.SMR[6].Reset,0,1)BTD(Port_Data.Data_Transfer[65],4,Hub.Write.SMR[5].Reset,0,1)BTD(Port_Data.Data_Transfer[65],3,Hub.Write.SMR[4].Reset,0,1)BTD(Port_Data.Data_Transfer[65],2,Hub.Write.SMR[3].Reset,0,1)BTD(Port_Data.Data_Transfer[65],1,Hub.Write.SMR[2].Reset,0,1)BTD(Port_Data.Data_Transfer[65],0,Hub.Write.SMR[1].Reset,0,1)OTU(Port_Data.Port_Read.[Port])OTL(Control.25);
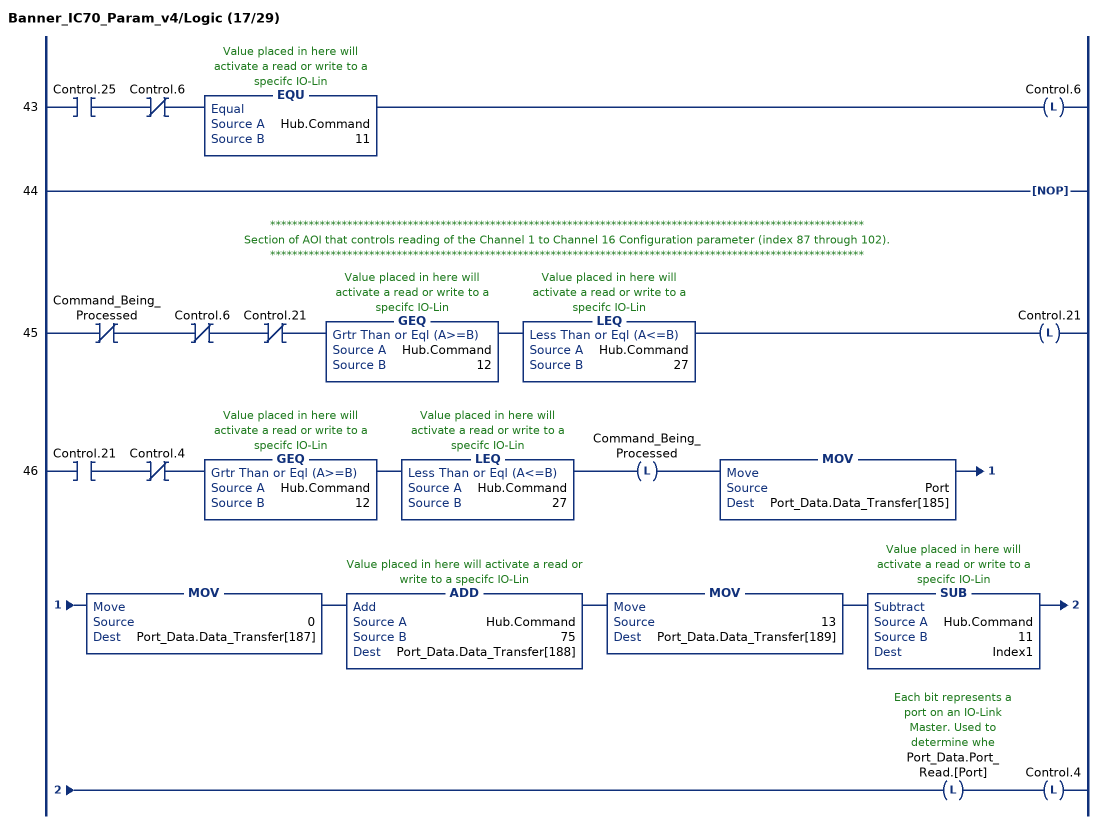
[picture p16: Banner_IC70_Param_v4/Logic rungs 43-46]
   43: XIC(Control.25)XIO(Control.6)EQU(Hub.Command,11)OTL(Control.6);
   44: NOP();
   // ************************************************************************************************************
   // Section of AOI that controls reading of the Channel 1 to Channel 16 Configuration parameter (index 87 through 102).
   // ************************************************************************************************************
   45: XIO(Command_Being_Processed)XIO(Control.6)XIO(Control.21)GEQ(Hub.Command,12)LEQ(Hub.Command,27)OTL(Control.21);
   46: XIC(Control.21)XIO(Control.4)GEQ(Hub.Command,12)LEQ(Hub.Command,27)OTL(Command_Being_Processed)MOV(Port,Port_Data.Data_Transfer[185])MOV(0,Port_Data.Data_Transfer[187])ADD(Hub.Command,75,Port_Data.Data_Transfer[188])MOV(13,Port_Data.Data_Transfer[189])SUB(Hub.Command,11,Index1)OTL(Port_Data.Port_Read.[Port])OTL(Control.4);
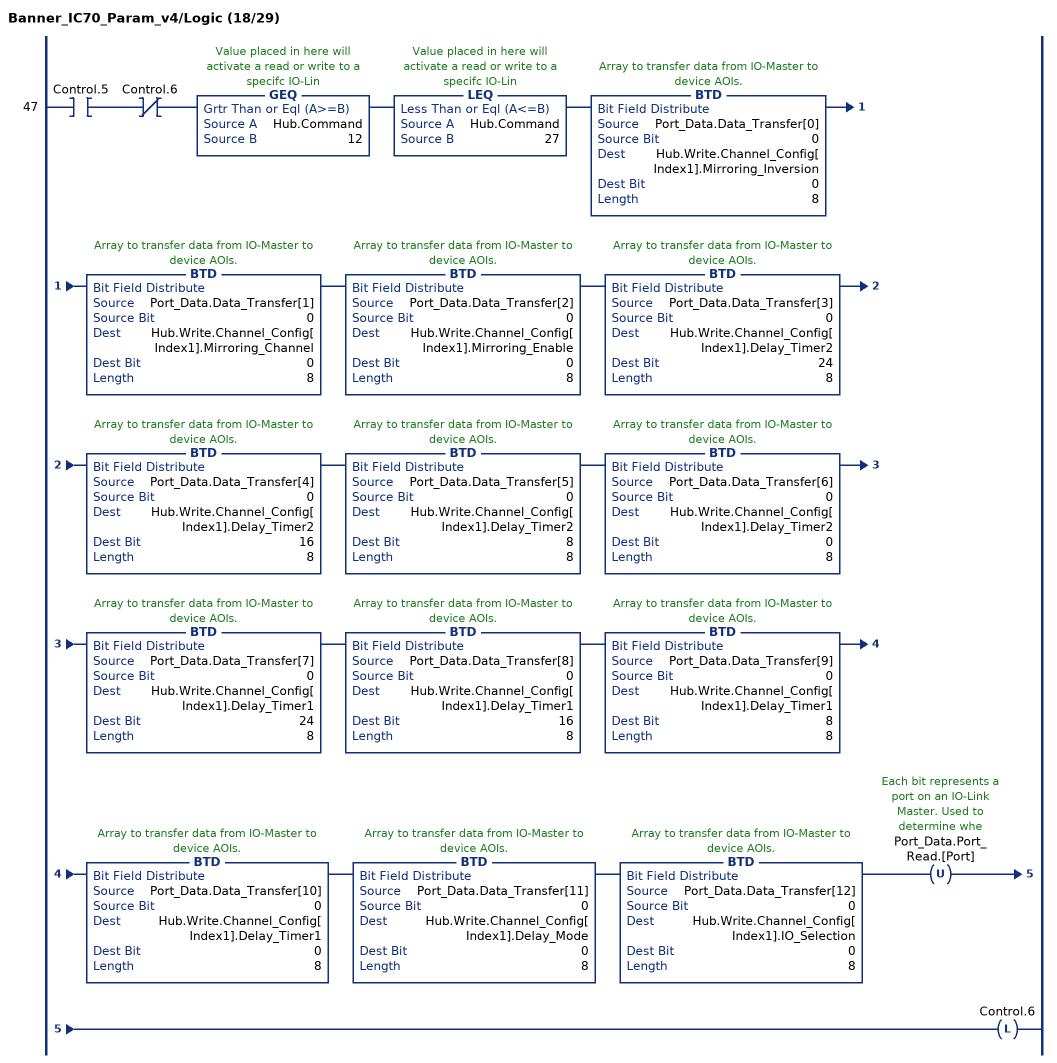
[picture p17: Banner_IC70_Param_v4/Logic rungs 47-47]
   47: XIC(Control.5)XIO(Control.6)GEQ(Hub.Command,12)LEQ(Hub.Command,27)BTD(Port_Data.Data_Transfer[0],0,Hub.Write.Channel_Config[Index1].Mirroring_Inversion,0,8)BTD(Port_Data.Data_Transfer[1],0,Hub.Write.Channel_Config[Index1].Mirroring_Channel,0,8)BTD(Port_Data.Data_Transfer[2],0,Hub.Write.Channel_Config[Index1].Mirroring_Enable,0,8)BTD(Port_Data.Data_Transfer[3],0,Hub.Write.Channel_Config[Index1].Delay_Timer2,24,8)BTD(Port_Data.Data_Transfer[4],0,Hub.Write.Channel_Config[Index1].Delay_Timer2,16,8)BTD(Port_Data.Data_Transfer[5],0,Hub.Write.Channel_Config[Index1].Delay_Timer2,8,8)BTD(Port_Data.Data_Transfer[6],0,Hub.Write.Channel_Config[Index1].Delay_Timer2,0,8)BTD(Port_Data.Data_Transfer[7],0,Hub.Write.Channel_Config[Index1].Delay_Timer1,24,8)BTD(Port_Data.Data_Transfer[8],0,Hub.Write.Channel_Config[Index1].Delay_Timer1,16,8)BTD(Port_Data.Data_Transfer[9],0,Hub.Write.Channel_Config[Index1].Delay_Timer1,8,8)BTD(Port_Data.Data_Transfer[10],0,Hub.Write.Channel_Config[Index1].Delay_Timer1,0,8)BTD(Port_Data.Data_Transfer[11],0,Hub.Write.Channel_Config[Index1].Delay_Mode,0,8)BTD(Port_Data.Data_Transfer[12],0,Hub.Write.Channel_Config[Index1].IO_Selection,0,8)OTU(Port_Data.Port_Read.[Port])OTL(Control.6);
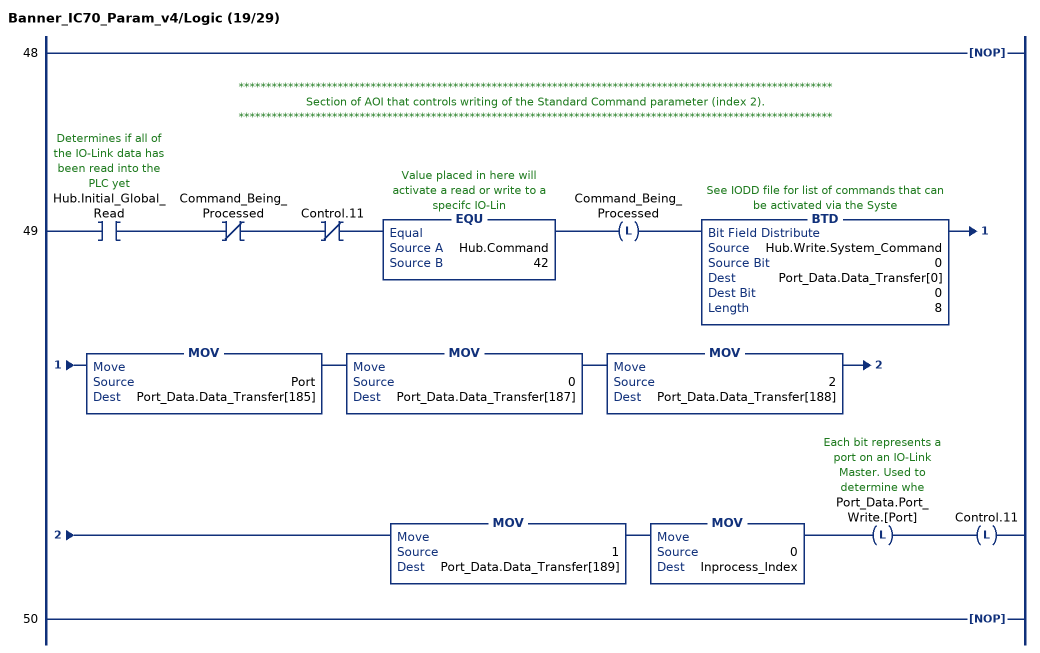
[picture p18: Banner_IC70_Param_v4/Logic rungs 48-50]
   48: NOP();
   // ************************************************************************************************************
   // Section of AOI that controls writing of the Standard Command parameter (index 2).
   // ************************************************************************************************************
   49: XIC(Hub.Initial_Global_Read)XIO(Command_Being_Processed)XIO(Control.11)EQU(Hub.Command,42)OTL(Command_Being_Processed)BTD(Hub.Write.System_Command,0,Port_Data.Data_Transfer[0],0,8)MOV(Port,Port_Data.Data_Transfer[185])MOV(0,Port_Data.Data_Transfer[187])MOV(2,Port_Data.Data_Transfer[188])MOV(1,Port_Data.Data_Transfer[189])MOV(0,Inprocess_Index)OTL(Port_Data.Port_Write.[Port])OTL(Control.11);
   50: NOP();
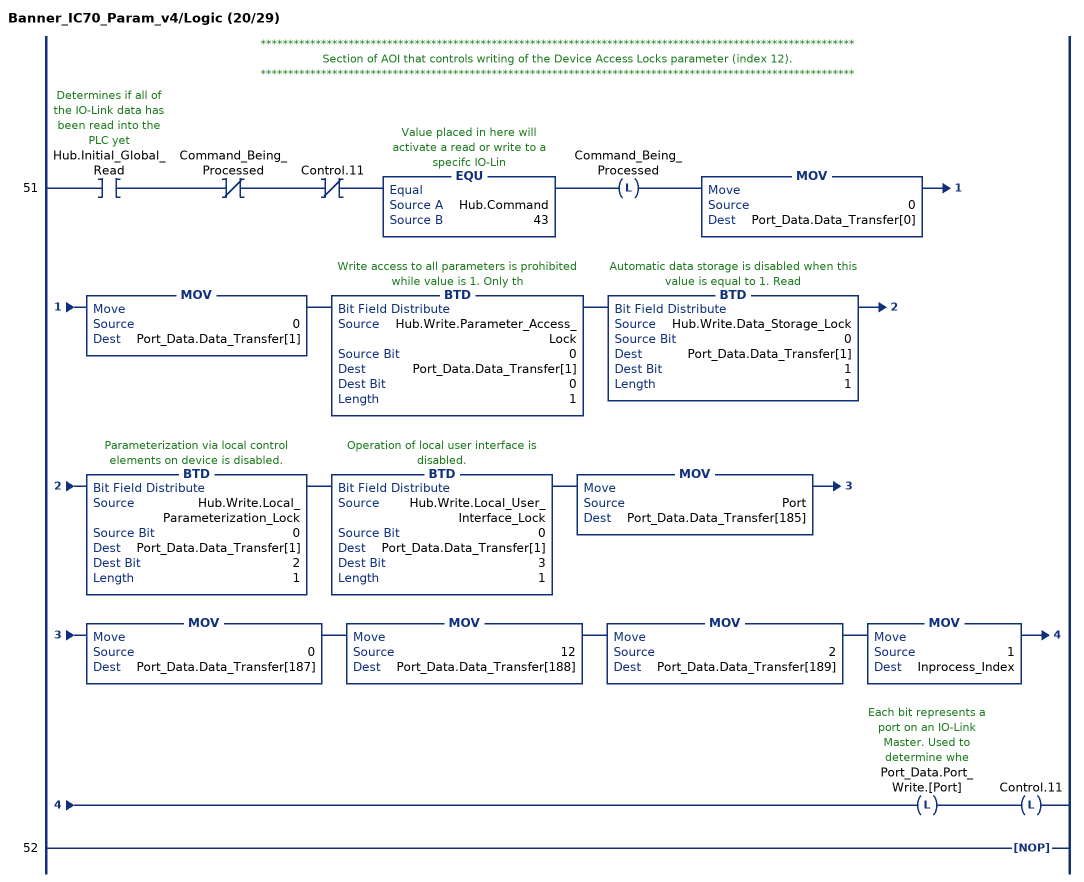
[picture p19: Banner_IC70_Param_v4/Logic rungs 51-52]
   // ************************************************************************************************************
   // Section of AOI that controls writing of the Device Access Locks parameter (index 12).
   // ************************************************************************************************************
   51: XIC(Hub.Initial_Global_Read)XIO(Command_Being_Processed)XIO(Control.11)EQU(Hub.Command,43)OTL(Command_Being_Processed)MOV(0,Port_Data.Data_Transfer[0])MOV(0,Port_Data.Data_Transfer[1])BTD(Hub.Write.Parameter_Access_Lock,0,Port_Data.Data_Transfer[1],0,1)BTD(Hub.Write.Data_Storage_Lock,0,Port_Data.Data_Transfer[1],1,1)BTD(Hub.Write.Local_Parameterization_Lock,0,Port_Data.Data_Transfer[1],2,1)BTD(Hub.Write.Local_User_Interface_Lock,0,Port_Data.Data_Transfer[1],3,1)MOV(Port,Port_Data.Data_Transfer[185])MOV(0,Port_Data.Data_Transfer[187])MOV(12,Port_Data.Data_Transfer[188])MOV(2,Port_Data.Data_Transfer[189])MOV(1,Inprocess_Index)OTL(Port_Data.Port_Write.[Port])OTL(Control.11);
   52: NOP();
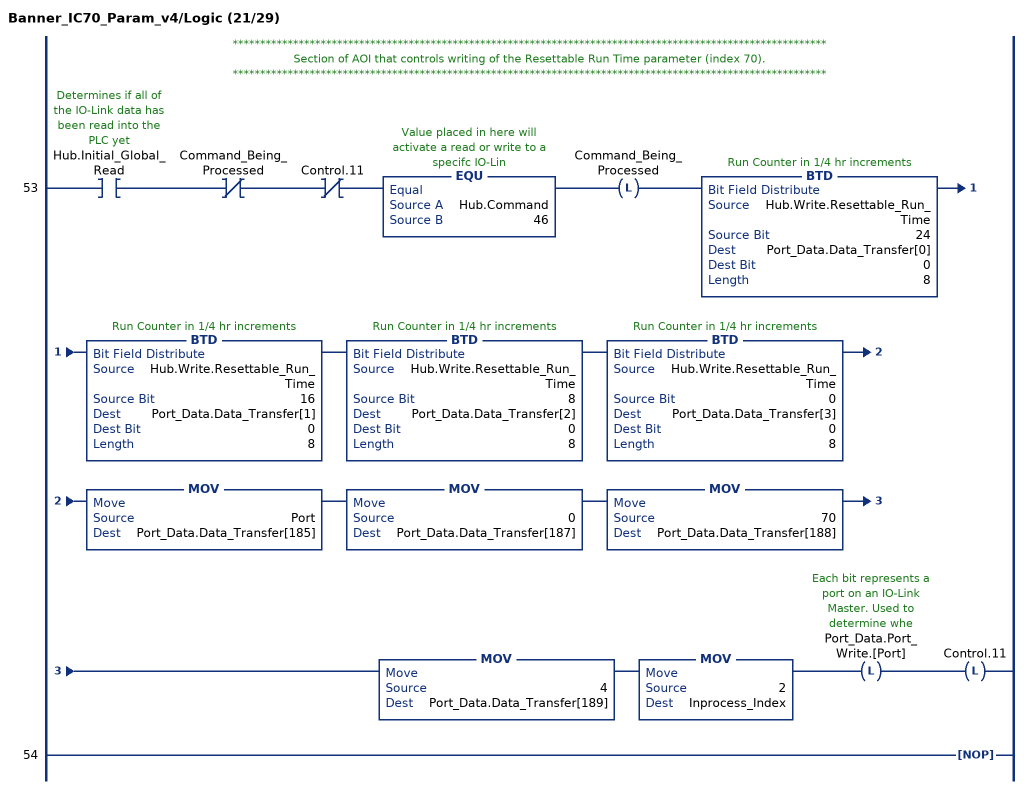
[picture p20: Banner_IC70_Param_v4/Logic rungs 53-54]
   // ************************************************************************************************************
   // Section of AOI that controls writing of the Resettable Run Time parameter (index 70).
   // ************************************************************************************************************
   53: XIC(Hub.Initial_Global_Read)XIO(Command_Being_Processed)XIO(Control.11)EQU(Hub.Command,46)OTL(Command_Being_Processed)BTD(Hub.Write.Resettable_Run_Time,24,Port_Data.Data_Transfer[0],0,8)BTD(Hub.Write.Resettable_Run_Time,16,Port_Data.Data_Transfer[1],0,8)BTD(Hub.Write.Resettable_Run_Time,8,Port_Data.Data_Transfer[2],0,8)BTD(Hub.Write.Resettable_Run_Time,0,Port_Data.Data_Transfer[3],0,8)MOV(Port,Port_Data.Data_Transfer[185])MOV(0,Port_Data.Data_Transfer[187])MOV(70,Port_Data.Data_Transfer[188])MOV(4,Port_Data.Data_Transfer[189])MOV(2,Inprocess_Index)OTL(Port_Data.Port_Write.[Port])OTL(Control.11);
   54: NOP();
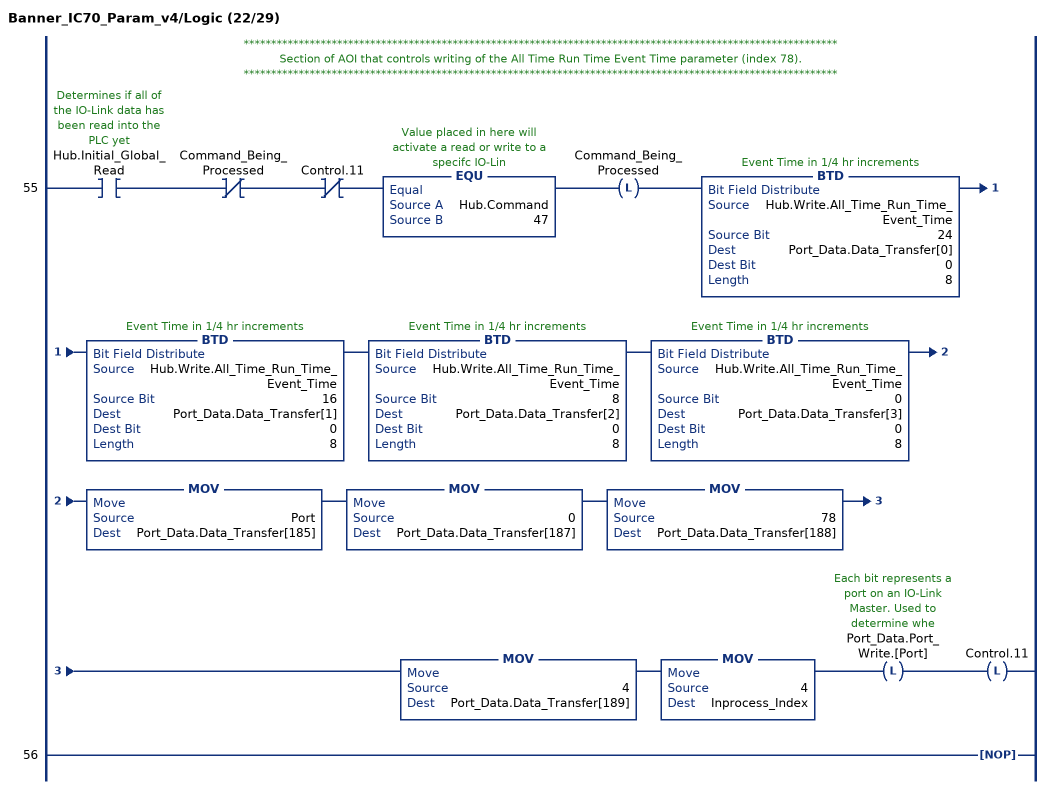
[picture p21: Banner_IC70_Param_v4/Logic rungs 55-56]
   // ************************************************************************************************************
   // Section of AOI that controls writing of the All Time Run Time Event Time parameter (index 78).
   // ************************************************************************************************************
   55: XIC(Hub.Initial_Global_Read)XIO(Command_Being_Processed)XIO(Control.11)EQU(Hub.Command,47)OTL(Command_Being_Processed)BTD(Hub.Write.All_Time_Run_Time_Event_Time,24,Port_Data.Data_Transfer[0],0,8)BTD(Hub.Write.All_Time_Run_Time_Event_Time,16,Port_Data.Data_Transfer[1],0,8)BTD(Hub.Write.All_Time_Run_Time_Event_Time,8,Port_Data.Data_Transfer[2],0,8)BTD(Hub.Write.All_Time_Run_Time_Event_Time,0,Port_Data.Data_Transfer[3],0,8)MOV(Port,Port_Data.Data_Transfer[185])MOV(0,Port_Data.Data_Transfer[187])MOV(78,Port_Data.Data_Transfer[188])MOV(4,Port_Data.Data_Transfer[189])MOV(4,Inprocess_Index)OTL(Port_Data.Port_Write.[Port])OTL(Control.11);
   56: NOP();
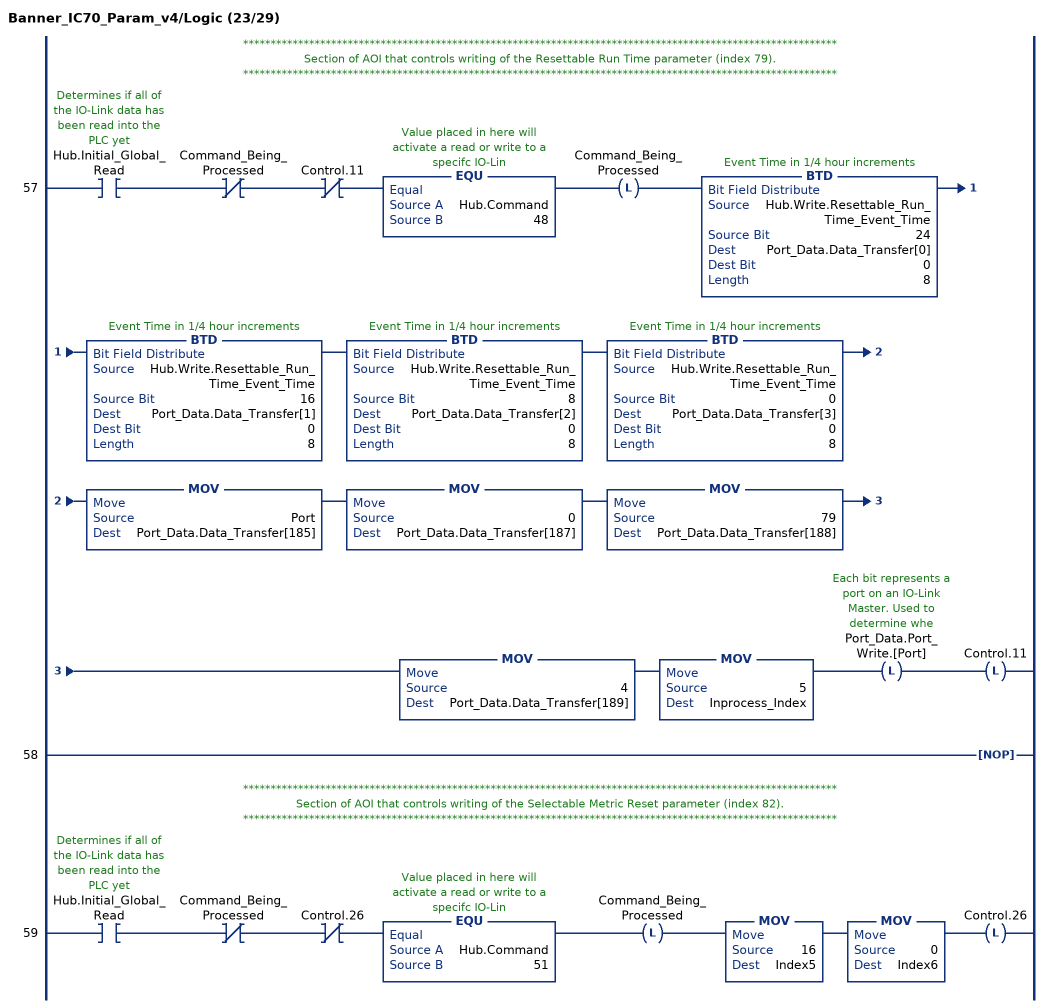
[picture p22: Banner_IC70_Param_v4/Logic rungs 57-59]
   // ************************************************************************************************************
   // Section of AOI that controls writing of the Resettable Run Time parameter (index 79).
   // ************************************************************************************************************
   57: XIC(Hub.Initial_Global_Read)XIO(Command_Being_Processed)XIO(Control.11)EQU(Hub.Command,48)OTL(Command_Being_Processed)BTD(Hub.Write.Resettable_Run_Time_Event_Time,24,Port_Data.Data_Transfer[0],0,8)BTD(Hub.Write.Resettable_Run_Time_Event_Time,16,Port_Data.Data_Transfer[1],0,8)BTD(Hub.Write.Resettable_Run_Time_Event_Time,8,Port_Data.Data_Transfer[2],0,8)BTD(Hub.Write.Resettable_Run_Time_Event_Time,0,Port_Data.Data_Transfer[3],0,8)MOV(Port,Port_Data.Data_Transfer[185])MOV(0,Port_Data.Data_Transfer[187])MOV(79,Port_Data.Data_Transfer[188])MOV(4,Port_Data.Data_Transfer[189])MOV(5,Inprocess_Index)OTL(Port_Data.Port_Write.[Port])OTL(Control.11);
   58: NOP();
   // ************************************************************************************************************
   // Section of AOI that controls writing of the Selectable Metric Reset parameter (index 82).
   // ************************************************************************************************************
   59: XIC(Hub.Initial_Global_Read)XIO(Command_Being_Processed)XIO(Control.26)EQU(Hub.Command,51)OTL(Command_Being_Processed)MOV(16,Index5)MOV(0,Index6)OTL(Control.26);
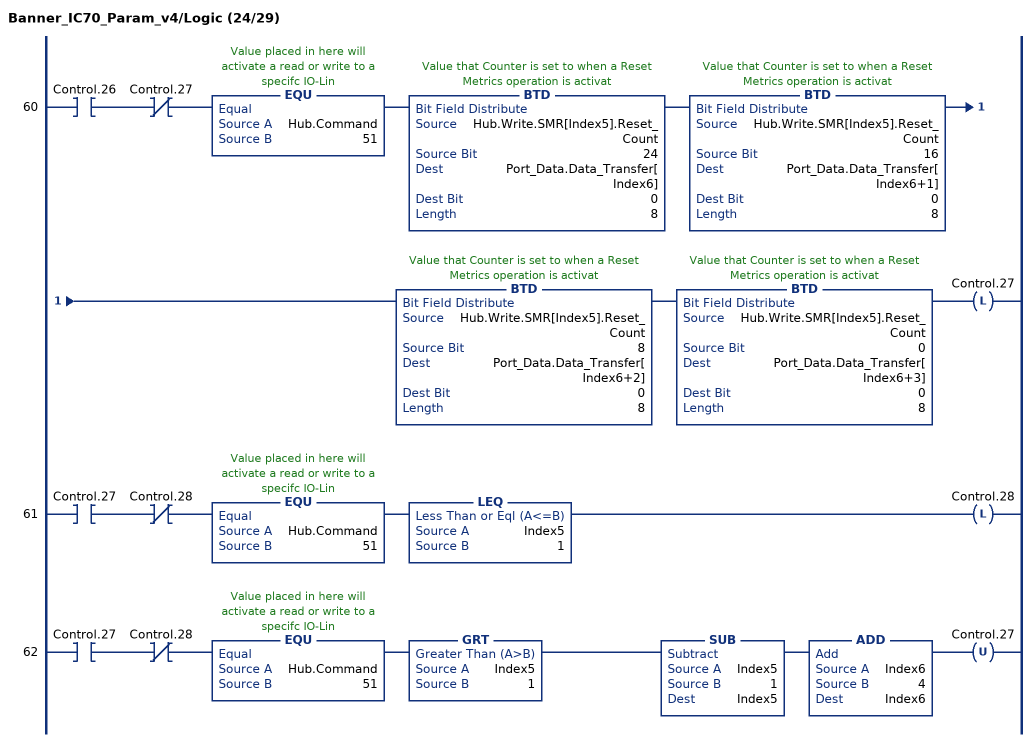
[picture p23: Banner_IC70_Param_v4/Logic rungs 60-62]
   60: XIC(Control.26)XIO(Control.27)EQU(Hub.Command,51)BTD(Hub.Write.SMR[Index5].Reset_Count,24,Port_Data.Data_Transfer[Index6],0,8)BTD(Hub.Write.SMR[Index5].Reset_Count,16,Port_Data.Data_Transfer[Index6+1],0,8)BTD(Hub.Write.SMR[Index5].Reset_Count,8,Port_Data.Data_Transfer[Index6+2],0,8)BTD(Hub.Write.SMR[Index5].Reset_Count,0,Port_Data.Data_Transfer[Index6+3],0,8)OTL(Control.27);
   61: XIC(Control.27)XIO(Control.28)EQU(Hub.Command,51)LEQ(Index5,1)OTL(Control.28);
   62: XIC(Control.27)XIO(Control.28)EQU(Hub.Command,51)GRT(Index5,1)SUB(Index5,1,Index5)ADD(Index6,4,Index6)OTU(Control.27);
